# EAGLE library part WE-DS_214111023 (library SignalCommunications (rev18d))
WE-DS D-SUB-Filter Solder Cup Characteristics Easy soldering, even for small strand cross sections Standard type filtered with 1000 pF High attenuation: max. ≥ 40 dB @ 180 MHz Choice of UNC 4/40 or through hole Rated voltage: 100 VDC Rated current @ 20 ºC: 5 A Withstand voltage: 250 VRMS Insulation resistance: min. 1000 MΩ Operating temperature: –55 ºC to +125 ºC Applications Filtering of interfaces External connection to -printer -sensor -display Details see: http://katalog.we-online.de/en/pbs/D-SUB-FILTER-SOLDER-CUP/210613023 2016 (C) Wurth Elektronik
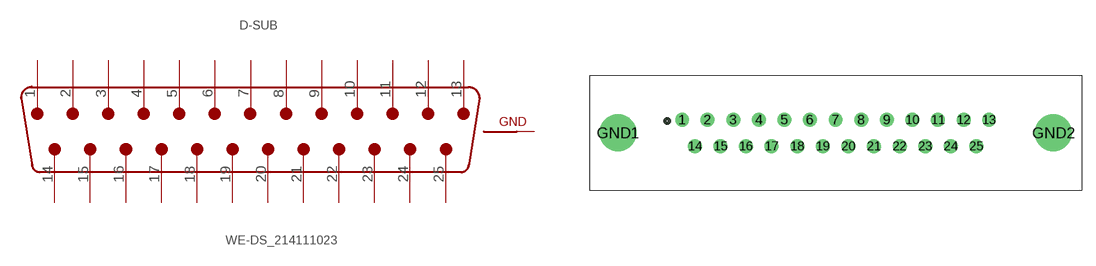
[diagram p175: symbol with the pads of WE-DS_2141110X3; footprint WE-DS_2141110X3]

Designator prefix D-SUB

## WE-DS_214111023 (WE-NUMBER: 214111023/25pins_male)  [WE-DS_2141110X3]
1  1  pas
2  2  pas
3  3  pas
4  4  pas
5  5  pas
6  6  pas
7  7  pas
8  8  pas
9  9  pas
10  10  pas
11  11  pas
12  12  pas
13  13  pas
14  14  pas
15  15  pas
16  16  pas
17  17  pas
18  18  pas
19  19  pas
20  20  pas
21  21  pas
22  22  pas
23  23  pas
24  24  pas
25  25  pas
GND1  GND  pwr
GND2  GND  pwr

## Footprint WE-DS_2141110X3 (pad centres in mm)
drill 1: 1 -16.56,1.42; 2 -13.82,1.42; 3 -11.05,1.42; 4 -8.28,1.42; 5 -5.54,1.42; 6 -2.77,1.42; 7 0,1.42; 8 2.77,1.42; 9 5.54,1.42; 10 8.28,1.42; 11 11.05,1.42; 12 13.82,1.42; 13 16.56,1.42; 14 -15.19,-1.42; 15 -12.42,-1.42; 16 -9.68,-1.42; 17 -6.91,-1.42; 18 -4.14,-1.42; 19 -1.38,-1.42; 20 1.38,-1.42; 21 4.14,-1.42; 22 6.91,-1.42; 23 9.68,-1.42; 24 12.42,-1.42; 25 15.19,-1.42
drill 3: GND1 -23.5,0; GND2 23.5,0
